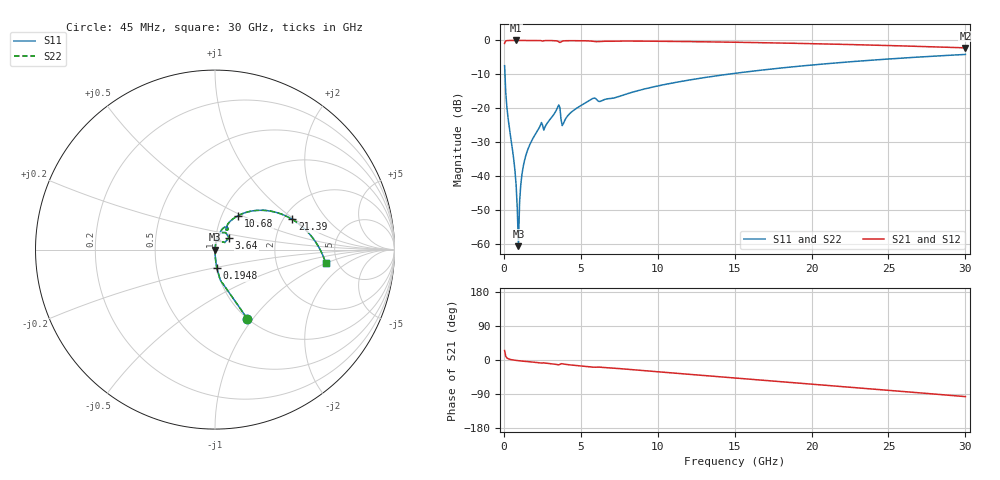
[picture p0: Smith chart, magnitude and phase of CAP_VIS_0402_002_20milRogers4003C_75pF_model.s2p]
! S-parameter model data by Modelithics Inc.  support@modelithics.com  813-866-6335  Tampa FL USA
! S-Parameter data specifications:
! Substrate: 20-mil Rogers 4003C, substrate thickness, H=0.508mm, Dielectric constant, Er=3.75
! PCB Mounting Pad Footprint: Pad width, PadW=0.50mm , Pad length, PadL=0.50mm , Pad gap, PadG (edge-to-edge)=0.40mm , Reference planes=1.4mm apart
! Created Wed Nov 18 12:56:53 2015
# hz S ma R 50
! 2 Port Network Data from SP1.SP block
! freq  magS11  angS11  magS21  angS21  magS12  angS12  magS22  angS22
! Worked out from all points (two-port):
!   401 points, 45 MHz to 30 GHz, reference 50 ohm
!   highest |S21| = -0.01 dB at 793.9 MHz (marker M1); lowest = -2.2 dB at 30 GHz (marker M2)
!   |S21| within 3 dB of the highest: start of sweep to end of sweep
!   lowest |S11| = -60.7 dB at 943.6 MHz (marker M3), VSWR 1.00, Z = 50.1 + j0.0511 ohm
!   |S11| at or under -10 dB: 69.19 MHz to 14.51 GHz (14.44 GHz wide, 198 % of centre)
!   |S22| runs from -60.7 to -4.1 dB; largest |S21 - S12| = 0
!   S11 on the Smith chart (normalised r, x): 45 MHz: 1.00, -0.94; 194.8 MHz: 1.00, -0.21; 3.64 GHz: 1.16, +0.16; 10.68 GHz: 1.19, +0.48; 21.39 GHz: 2.23, +0.95; 30 GHz: 4.03, -1.00
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4.5e7  0.4243 -65.0  0.9053 25.0  0.9053 25.0  0.4243 -65.0
1.94775e8  0.1032 -84.2  0.9943 5.6  0.9943 5.6  0.1032 -84.2
6.441e8  0.01722 -88.1  0.9992 -0.2  0.9992 -0.2  0.01722 -88.1
7.93875e8  0.007397 -85.7  0.9992 -1.1  0.9992 -1.1  0.007397 -85.7
9.4365e8  0.0009278 33.4  0.9992 -1.8  0.9992 -1.8  0.0009278 33.4
1.093425e9  0.007348 81.2  0.9991 -2.5  0.9991 -2.5  0.007348 81.2
1.168312e9  0.01044 82.6  0.9991 -2.8  0.9991 -2.8  0.01044 82.6
1.318088e9  0.01624 83.4  0.9989 -3.4  0.9989 -3.4  0.01624 83.4
1.692525e9  0.02945 83.1  0.9985 -4.9  0.9985 -4.9  0.02945 83.1
2.366512e9  0.05579 78.8  0.9949 -7.6  0.9949 -7.6  0.05579 78.8
2.74095e9  0.05687 78.7  0.9954 -8.4  0.9954 -8.4  0.05687 78.7
3.489825e9  0.1032 67.4  0.9765 -12.4  0.9765 -12.4  0.1032 67.4
3.6396e9  0.1027 40.7  0.9337 -11.5  0.9337 -11.5  0.1027 40.7
3.864262e9  0.05923 64.9  0.9834 -10.6  0.9834 -10.6  0.05923 64.9
5.062462e9  0.1116 72.0  0.9896 -15.9  0.9896 -15.9  0.1116 72.0
1.007992e10  0.2152 57.5  0.9722 -31.4  0.9722 -31.4  0.2152 57.5
1.067902e10  0.2293 55.7  0.9692 -33.3  0.9692 -33.3  0.2293 55.7
1.50225e10  0.3276 41.9  0.9407 -47.4  0.9407 -47.4  0.3276 41.9
2.003996e10  0.4346 25.8  0.8961 -63.7  0.8961 -63.7  0.4346 25.8
2.138794e10  0.4621 21.4  0.8822 -68.1  0.8822 -68.1  0.4621 21.4
2.505742e10  0.5336 9.4  0.8406 -80.2  0.8406 -80.2  0.5336 9.4
3e10  0.6219 -7.0  0.7773 -96.6  0.7773 -96.6  0.6219 -7.0
